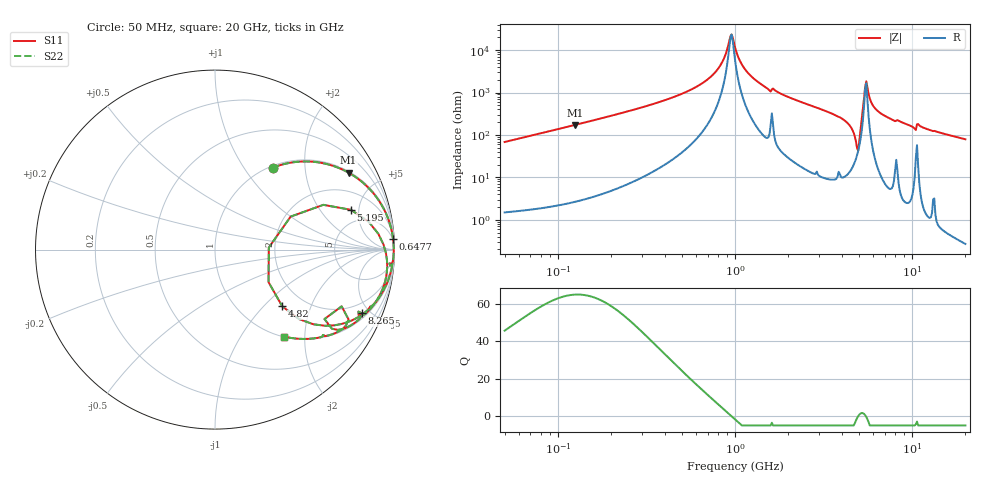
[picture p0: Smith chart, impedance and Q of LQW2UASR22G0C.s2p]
!Murata Part Number: LQW2UASR22G0C
!These Parameters are Measured in Series Mode Connection
!  o--[Z]--o
!Port1  Port2
!  o-------o
!Freq. Start=50[MHz] Stop=20[GHz], 401[Steps]
# Hz S RI R 50
!Freq.(Hz) S11(Real) S11(Imag) S21(Real) S21(Imag) S12(Real) S12(Imag) S22(Real) S22(Imag)
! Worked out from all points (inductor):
!   401 points, 50 MHz to 20 GHz, reference 50 ohm
!   read as one part in series: L = 216 nH near 51.52 MHz
!   highest Q = 65.1 at 124.7 MHz (marker M1), where L = 219 nH
!   self-resonance near 941.8 MHz
!   S11 on the Smith chart (normalised r, x): 50 MHz: 1.03, +1.36; 647.7 MHz: 3, +32; 4.82 GHz: 1.55, -1.29; 5.195 GHz: 3.49, +4.10; 8.265 GHz: 1.29, -4.46; 20 GHz: 1.01, -1.58
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5e7  0.321 0.4561  0.679 -0.4561  0.679 -0.4561  0.321 0.4561
1.246764e8  0.744 0.4288  0.256 -0.4288  0.256 -0.4288  0.744 0.4288
1.364002e8  0.7773 0.4085  0.2227 -0.4085  0.2227 -0.4085  0.7773 0.4085
3.721004e8  0.9682 0.1623  0.0318 -0.1623  0.0318 -0.1623  0.9682 0.1623
6.476653e8  0.992 0.061  0.00804 -0.061  0.00804 -0.061  0.992 0.061
8.230629e8  0.9952 0.0229  0.00478 -0.0229  0.00478 -0.0229  0.9952 0.0229
9.418449e8  0.9957 0.00204  0.00425 -0.00204  0.00425 -0.00204  0.9957 0.00204
1e9  0.9957 -0.00726  0.0043 0.00726  0.0043 0.00726  0.9957 -0.00726
1.110545e9  0.9952 -0.0237  0.00484 0.0237  0.00484 0.0237  0.9952 -0.0237
1.329223e9  0.9928 -0.053  0.00722 0.053  0.00722 0.053  0.9928 -0.053
2.728004e9  0.9537 -0.1975  0.0463 0.1975  0.0463 0.1975  0.9537 -0.1975
4.149438e9  0.8185 -0.3629  0.1815 0.3629  0.1815 0.3629  0.8185 -0.3629
4.608136e9  0.6141 -0.4244  0.3859 0.4244  0.3859 0.4244  0.6141 -0.4244
4.81993e9  0.3748 -0.3161  0.6252 0.3161  0.6252 0.3161  0.3748 -0.3161
4.966507e9  0.2998 0.0116  0.7002 -0.0116  0.7002 -0.0116  0.2998 0.0116
5.194772e9  0.757 0.2217  0.243 -0.2217  0.243 -0.2217  0.757 0.2217
5.352748e9  0.9097 0.0886  0.0903 -0.0886  0.0903 -0.0886  0.9097 0.0886
5.515528e9  0.9528 -0.0214  0.0472 0.0214  0.0472 0.0214  0.9528 -0.0214
6.125241e9  0.9382 -0.2081  0.0618 0.2081  0.0618 0.2081  0.9382 -0.2081
7.442007e9  0.8554 -0.341  0.1446 0.341  0.1446 0.341  0.8554 -0.341
8.264682e9  0.8179 -0.3546  0.1821 0.3546  0.1821 0.3546  0.8179 -0.3546
2e10  0.3845 -0.4848  0.6155 0.4848  0.6155 0.4848  0.3845 -0.4848
